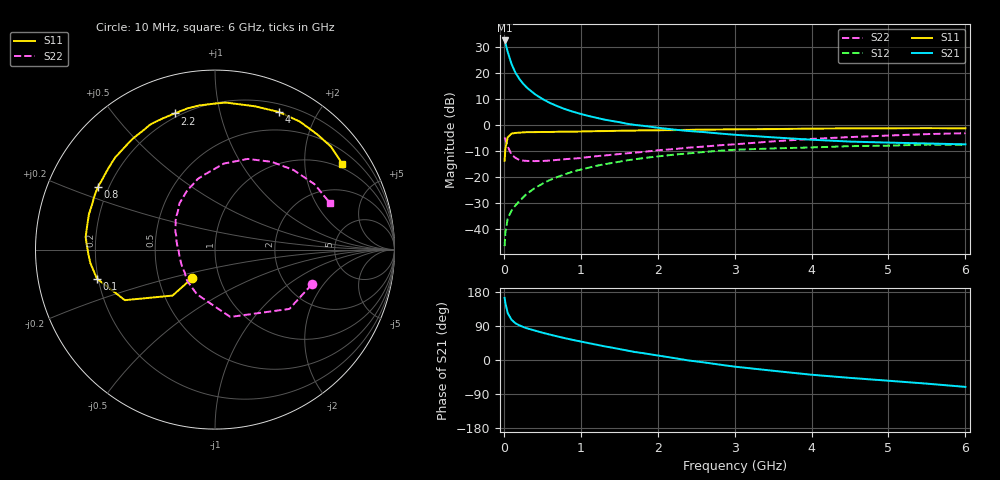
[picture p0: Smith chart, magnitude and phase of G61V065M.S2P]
! SIEMENS Small Signal Semiconductors
! BFG193
! Si NPN RF Bipolar Junction Transistor in SOT223
! VCE = 1 V  IC = 65 mA
! Common Emitter S-Parameters:  August  1996
# GHz  S  MA  R  50
!  f  S11  S21  S12  S22
! GHz  MAG  ANG  MAG  ANG  MAG  ANG  MAG  ANG
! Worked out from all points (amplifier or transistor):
!   36 points, 10 MHz to 6 GHz, reference 50 ohm
!   highest |S21| = 32.4 dB at 10 MHz (marker M1)
!   |S21| within 3 dB of that: start of sweep to 38.17 MHz
!   unconditionally stable (mu >= 1): start of sweep to 19.46 MHz; 139.3 MHz to end of sweep
!   at 250 MHz: K = 1.15, MAG = 19.5 dB, |S12| = -27.8 dB
!   at 1.4 GHz: K = 1.19, MAG = 5.5 dB, |S12| = -14.7 dB
!   at 6 GHz: K = 1.07, MAG = -1.5 dB, |S12| = -7.7 dB
!   S11 on the Smith chart (normalised r, x): 10 MHz: 0.74, -0.25; 100 MHz: 0.19, -0.12; 800 MHz: 0.16, +0.24; 2.2 GHz: 0.18, +0.73; 4 GHz: 0.28, +1.53; 6 GHz: 0.85, +3.04
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0.01  0.2047 -128.8  41.54 164.0  0.0047 69.8  0.5731 -19.8
0.02  0.3485 -132.7  37.41 150.5  0.0086 64.7  0.53 -38.6
0.05  0.5757 -150.7  25.14 123.9  0.0159 53.9  0.3847 -77.2
0.1  0.6775 -166.2  14.66 106.2  0.0226 56.2  0.2688 -111.9
0.15  0.6988 -173.9  10.04 97.0  0.0283 58.6  0.233 -131.8
0.2  0.7071 -178.5  7.68 91.6  0.0342 62.0  0.2118 -143.0
0.25  0.715 177.9  6.164 87.3  0.0406 63.4  0.2056 -153.3
0.3  0.7242 174.5  5.17 83.7  0.0477 64.9  0.2031 -159.1
0.4  0.7244 169.6  3.906 77.9  0.0608 65.0  0.2015 -169.7
0.5  0.7296 164.4  3.141 72.1  0.0738 63.9  0.2022 -177.2
0.6  0.729 160.2  2.627 67.0  0.0876 63.0  0.2065 177.4
0.8  0.7395 151.9  1.989 57.3  0.1134 59.2  0.2197 167.6
1.1  0.7502 140.7  1.479 44.6  0.1503 52.9  0.2408 156.2
1.3  0.7585 133.5  1.266 36.4  0.1745 48.3  0.2575 148.4
1.6  0.7717 123.7  1.05 25.1  0.2081 40.4  0.2842 139.4
2.2  0.7912 106.5  0.814 5.6  0.2666 25.1  0.3412 121.4
2.8  0.8126 90.6  0.682 -12.1  0.3183 10.0  0.4051 103.7
3.5  0.8289 74.4  0.575 -28.4  0.3528 -8.3  0.4815 84.2
4  0.8453 65.1  0.518 -38.9  0.3682 -18.0  0.537 70.2
4.5  0.8555 56.5  0.477 -47.2  0.3898 -27.8  0.5824 57.1
5.5  0.864 41.6  0.439 -62.4  0.4174 -50.0  0.6635 33.3
6  0.8556 34.1  0.422 -71.0  0.4139 -62.5  0.6911 22.0
